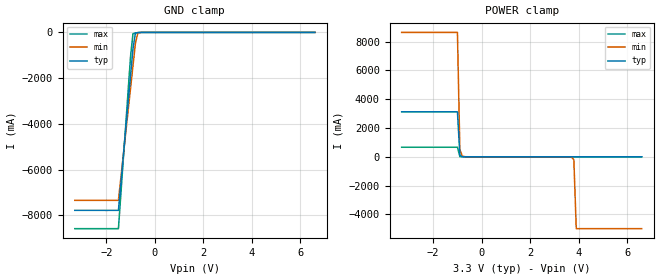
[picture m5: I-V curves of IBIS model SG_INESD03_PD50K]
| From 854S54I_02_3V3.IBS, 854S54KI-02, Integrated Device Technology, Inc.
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[Model]   SG_INESD03_PD50K
Model_type   Input
Polarity   Non-Inverting
Vinl = 0.8V
Vinh = 2.0V
|   typ   min   max
C_comp   2pF   1.5pF   2.5pF
|   typ   min   max
[Voltage range]  3.3V   3.135V   3.465V
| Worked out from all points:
|   GND clamp passes 1 mA (typ) near -0.54 V on its own axis
|   POWER clamp passes 1 mA (typ) near -0.71 V on its own axis
[GND_clamp]
|Voltage I(typ)   I(min)   I(max)
-3.3V     -7.788A    -7.349A    -8.588A
-1.5V     -7.788A    -7.349A    -8.588A
-1V       -1.886A    -2.44A     -1.044A
-900mV    -707.1mA   -1.46A     -57.39mA
-800mV    -35.57mA   -480.7mA   -24.35mA
-700mV    -6.978mA   -23.99mA   -13.24mA
-600mV    -2.058mA   -1.658mA   -4.859mA
6.6V      128.6uA    160.8uA    121.8uA
[POWER_clamp]
|Voltage   I(typ)   I(min)   I(max)
-3.3V     3.124A     8.649A     661.5mA
-1V       3.124A     8.649A     661.5mA
-900mV    134.8mA    492.4mA    8.633mA
-800mV    4.998mA    58.35mA    519.6uA
-600mV    119.1uA    404uA      77.42uA
3.7V      -33.68uA   -9.524mA   -4.372uA
3.8V      -368.1uA   -207.7mA   -6.375uA
3.9V      -2.221mA   -5A        -18.91uA
6.6V      -2.221mA   -5A        -18.91uA
